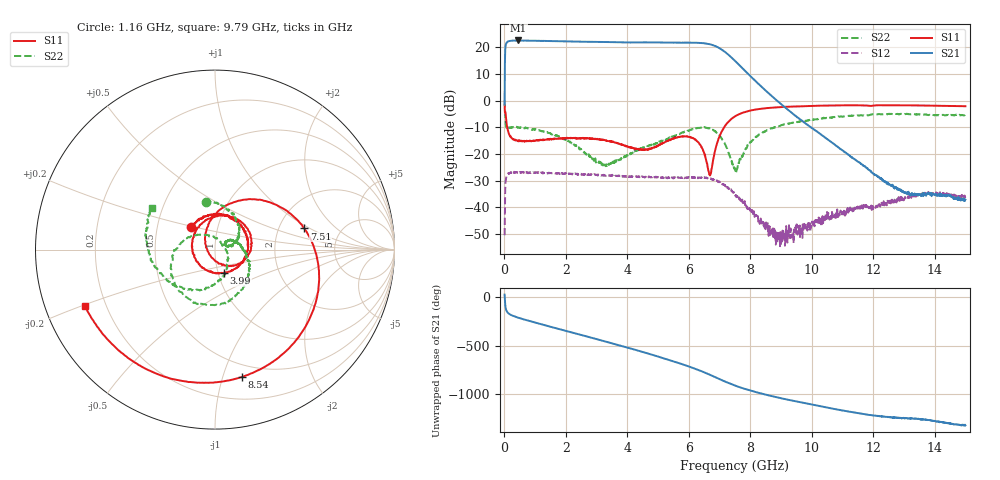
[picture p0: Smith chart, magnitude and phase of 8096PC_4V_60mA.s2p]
!Keysight Technologies,N5247B,US58420632,A.15.75.19
!Date: Wednesday, November 02, 2022 15:42:31
!Correction: S11(C  2-Port  )
!S21(C  2-Port  )
!S12(C  2-Port  )
!S22(C  2-Port  )
!S2P File: Measurements: S11, S21, S12, S22:
# Hz S  dB  R 50
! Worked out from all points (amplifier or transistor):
!   1500 points, 10 MHz to 15 GHz, reference 50 ohm
!   highest |S21| = 22.6 dB at 460 MHz (marker M1)
!   |S21| within 3 dB of that: 34.23 MHz to 7.014 GHz (6.98 GHz wide, 198 % of centre)
!   unconditionally stable (mu >= 1): 11.82 MHz to end of sweep
!   at 2.51 GHz: K = 1.17, MAG = 22.5 dB, |S12| = -27.8 dB
!   at 7.51 GHz: K = 3.96, MAG = 16.2 dB, |S12| = -35.4 dB
!   at 15 GHz: K = 596.16, MAG = -31.4 dB, |S12| = -35.8 dB
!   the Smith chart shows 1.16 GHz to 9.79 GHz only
!   S11 on the Smith chart (normalised r, x): 1.16 GHz: 0.74, +0.20; 3.99 GHz: 1.07, -0.29; 7.51 GHz: 2.77, +0.89; 8.54 GHz: 0.38, -1.15; 9.79 GHz: 0.12, -0.21
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1e7  -1.65 -33.1  -1.46 28.1  -50.47 8.6  0.15 -37.6
9e7  -9.70 -114.9  21.97 -150.0  -27.92 50.4  -10.34 -136.3
1.5e8  -12.45 -138.6  22.35 -169.6  -27.15 23.9  -10.11 -157.2
4.6e8  -15.24 178.8  22.60 148.6  -26.67 -22.6  -10.07 158.7
1.16e9  -14.65 136.2  22.44 85.2  -27.01 -80.8  -11.29 100.8
1.88e9  -14.22 93.0  22.28 24.0  -27.18 -133.8  -14.02 52.4
2.51e9  -14.04 55.4  22.11 -29.4  -27.80 179.6  -18.72 18.1
3.24e9  -14.70 1.6  22.01 -91.9  -28.13 124.2  -23.87 23.3
3.99e9  -17.05 -69.1  21.85 -157.5  -28.49 66.0  -20.41 35.8
4.47e9  -18.24 -133.4  21.89 159.3  -28.43 27.0  -17.85 19.5
5.01e9  -16.71 141.4  21.84 108.2  -28.80 -21.3  -15.64 -2.7
5.5e9  -14.30 77.4  21.78 59.9  -29.16 -62.6  -13.37 -27.7
6.07e9  -13.86 8.0  21.76 -0.7  -28.89 -114.6  -10.87 -67.5
6.37e9  -16.48 -33.7  21.68 -36.6  -28.86 -143.6  -10.13 -95.9
6.72e9  -27.36 179.9  21.08 -83.3  -29.13 173.7  -10.59 -138.2
7.1e9  -10.95 68.5  18.96 -137.6  -31.27 128.9  -14.69 165.1
7.51e9  -5.82 13.3  14.91 169.6  -35.37 81.9  -26.25 46.5
8.54e9  -2.78 -78.2  3.40 73.5  -47.58 26.7  -11.20 -127.9
9.79e9  -2.05 -156.3  -8.44 -12.0  -47.94 54.0  -7.52 146.1
1.001e10  -1.97 -168.6  -10.24 -26.2  -45.34 55.6  -7.01 133.3
1.251e10  -1.71 61.7  -31.16 -154.8  -38.39 -77.4  -4.93 -6.8
1.5e10  -2.07 -65.8  -37.11 119.8  -35.76 135.1  -5.44 -144.8
